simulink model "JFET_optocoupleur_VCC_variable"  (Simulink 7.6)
settings: Solver=ode15s  StartTime=0.0  StopTime=10.0  RelTol=1e-3
StopFcn:
  | close all, clc
  | load ID_Vcc_Variable.mat
  | delete *.mat
  | plotyy(x(1,:),x(2,:), x(1,:),x(3,:))
  | grid
  | title('Courant de drain ID et alimentation variable')
  | xlabel('temps')
libraries: fl_lib x10, elec_lib x5, nesl_utility x4

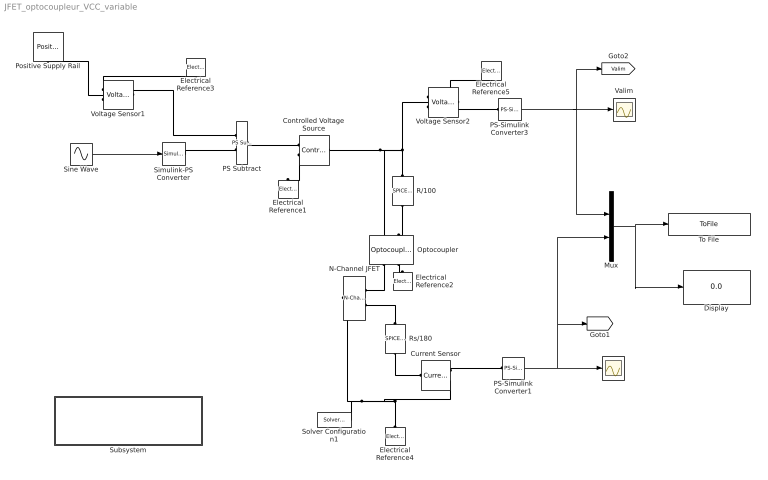
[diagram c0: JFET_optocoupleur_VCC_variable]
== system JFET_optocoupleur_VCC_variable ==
  Controlled Voltage Source : fl_lib/Electrical/Electrical Sources/Controlled Voltage Source  DialogController=NetworkEngine.DynNeDlgSource  SystemSampleTime=-1  i_Log=off  v_Log=off  LocalVarNames=|i|v  LocalVarDescs=|i|v  LocalVarLogging=[0 0]
  Current Sensor : fl_lib/Electrical/Electrical Sensors/Current Sensor  DialogController=NetworkEngine.DynNeDlgSource  SystemSampleTime=-1  i1_Log=off  v1_Log=off  LocalVarNames=|i1|v1  LocalVarDescs=|i1|v1  LocalVarLogging=[0 0]
  Display : Display
  Electrical Reference{1..5} (5 alike) : fl_lib/Electrical/Electrical Elements/Electrical Reference  DialogController=NetworkEngine.DynNeDlgSource  SystemSampleTime=-1  i_Log=off  LocalVarNames=|i  LocalVarDescs=|i  LocalVarLogging=[]
  I : Scope
  Mux : Mux  Inputs=2
  N-Channel JFET : elec_lib/Semiconductor Devices/N-Channel JFET  DialogController=NetworkEngine.DynNeDlgSource  SystemSampleTime=-1  parameterization=1  Igss=-1 nA  Idss=17 mA  Idss_v="[  0 15 ] V"  ssig="[  3e+03 10 ] uS"  ssig_v="[  0 15 ] V"  Beta=1e-04 A/V^2  IS=1e-14 A  Tmeas=25 C  Vt0=-2 V  Lchannel=0 1/V  RS=0.1 Ohm  RD=0.1 Ohm  C_param=1  C_GS=3 pF  C_GD=1.5 pF  C_iss=4.5 pF  C_rss=1.5 pF  LocalVarLogging=[]
  Optocoupler : elec_lib/Semiconductor Devices/Optocoupler  DialogController=NetworkEngine.DynNeDlgSource  SystemSampleTime=-1  CTR=0.2  prmExp=1  I12="[  0.001 0.015 ] A"  V12="[  0.9 1.05 ] V"  RS=0.1 Ohm  IS=1e-10 A  Tmeas=25 C  ec=2  C_param=1  CJ0=5 pF  VJ=1 V  Mgrad=0.5  Vvec="[  0.1 10 100 ] V"  Cvec="[  3.5 1 0.4 ] pF"  FC=0.5  LocalVarLogging=[]
  PS Subtract : fl_lib/Physical Signals/Functions/PS Subtract  DialogController=NetworkEngine.DynNeDlgSource  SystemSampleTime=-1  LocalVarLogging=[]
  PS-Simulink Converter1 : nesl_utility/PS-Simulink Converter  DialogController=NetworkEngine.DynNeUtilDlgSource  SystemSampleTime=-1  PhysicalDomain=network_engine_domain  LeftPortType=input  RightPortType=output  SubClassName=ps_output  Unit=1  AffineConversion=off
  PS-Simulink Converter3 : nesl_utility/PS-Simulink Converter  DialogController=NetworkEngine.DynNeUtilDlgSource  SystemSampleTime=-1  PhysicalDomain=network_engine_domain  LeftPortType=input  RightPortType=output  SubClassName=ps_output  Unit=1  AffineConversion=off
  Positive Supply Rail : elec_lib/Sources/Positive Supply Rail  DialogController=NetworkEngine.DynNeDlgSource  SystemSampleTime=-1  v0=15 V  current_Log=off  voltage_Log=off  power_Log=off  LocalVarNames=|current|voltage|power  LocalVarDescs=|Current (A)|Voltage (V)|Power (W)  LocalVarLogging=[0 0 0]
  R/100 : elec_lib/Additional Components/SPICE-Compatible Components/Passive Devices/SPICE Resistor  DialogController=NetworkEngine.DynNeDlgSource  SystemSampleTime=-1  SCALE=1  R_param=1  R=100 Ohm  RSH=0 Ohm  LENGTH=1e-06 m  WIDTH=1e-06 m  NARROW=0 m  T_param=1  TC1=0 1/K  TC2=0 1/K^2  TOFFSET=0 K  TFIXED=300.15 K  TMEAS=300.15 K  LocalVarLogging=[]
  Rs/180 : elec_lib/Additional Components/SPICE-Compatible Components/Passive Devices/SPICE Resistor  DialogController=NetworkEngine.DynNeDlgSource  SystemSampleTime=-1  SCALE=1  R_param=1  R=180 Ohm  RSH=0 Ohm  LENGTH=1e-06 m  WIDTH=1e-06 m  NARROW=0 m  T_param=1  TC1=0 1/K  TC2=0 1/K^2  TOFFSET=0 K  TFIXED=300.15 K  TMEAS=300.15 K  LocalVarLogging=[]
  Simulink-PS Converter : nesl_utility/Simulink-PS Converter  DialogController=NetworkEngine.DynNeUtilDlgSource  SystemSampleTime=-1  PhysicalDomain=network_engine_domain  LeftPortType=input  RightPortType=output  SubClassName=ps_input  Unit=1  AffineConversion=off  InputFilterTimeConstant=.001  UdotUserProvided=0
  Sine Wave : Sin  Amplitude=2  SampleTime=0
  Solver Configuration1 : nesl_utility/Solver Configuration  DialogController=NetworkEngine.DynNeUtilDlgSource  SystemSampleTime=-1  PhysicalDomain=network_engine_domain  LeftPortType=input  RightPortType=generic  SubClassName=solver  Accelerate=off  Profile=off  ResidualTolerance=1e-9  MaxNonlinIter=12  MaxModeIter=2  DoFixedCost=off  UseLocalSampling=off  DoDC=off  LinearAlgebra=Sparse  LocalSolverSampleTime=.001  LocalSolverChoice=NE_BACKWARD_EULER_ADVANCER  UseLocalSolver=off
  Subsystem : Subsystem
  To File : ToFile  Filename=ID_Vcc_Variable  MatrixName=x
  Valim : Scope
  Voltage Sensor1 : fl_lib/Electrical/Electrical Sensors/Voltage Sensor  DialogController=NetworkEngine.DynNeDlgSource  SystemSampleTime=-1  i1_Log=off  v1_Log=off  LocalVarNames=|i1|v1  LocalVarDescs=|i1|v1  LocalVarLogging=[0 0]
  Voltage Sensor2 : fl_lib/Electrical/Electrical Sensors/Voltage Sensor  DialogController=NetworkEngine.DynNeDlgSource  SystemSampleTime=-1  i1_Log=off  v1_Log=off  LocalVarNames=|i1|v1  LocalVarDescs=|i1|v1  LocalVarLogging=[0 0]
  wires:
  Sine Wave/1 -> Simulink-PS Converter/1
  PS-Simulink Converter1/1 -> I/1, [I], Mux/2
  PS-Simulink Converter3/1 -> Valim/1, [Valim], Mux/1
  Mux/1 -> To File/1, Display/1
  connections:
  N-Channel JFET/LConn1 -- Solver Configuration1/RConn1 -- Electrical Reference4/LConn1 -- Current Sensor/RConn2
  Rs/180/LConn1 -- N-Channel JFET/RConn2
  Optocoupler/LConn1 -- Controlled Voltage Source/LConn1 -- R/100/LConn1 -- Voltage Sensor2/LConn1
  Optocoupler/RConn1 -- N-Channel JFET/RConn1
  Optocoupler/RConn2 -- Electrical Reference2/LConn1
  R/100/RConn1 -- Optocoupler/LConn2
  Simulink-PS Converter/RConn1 -- PS Subtract/LConn2
  PS Subtract/RConn1 -- Controlled Voltage Source/RConn1
  Rs/180/RConn1 -- Current Sensor/LConn1
  Current Sensor/RConn1 -- PS-Simulink Converter1/LConn1
  Controlled Voltage Source/RConn2 -- Electrical Reference1/LConn1
  Voltage Sensor2/RConn1 -- PS-Simulink Converter3/LConn1
  Voltage Sensor2/RConn2 -- Electrical Reference5/LConn1
  Voltage Sensor1/RConn1 -- PS Subtract/LConn1
  Voltage Sensor1/LConn1 -- Positive Supply Rail/RConn1
  Voltage Sensor1/RConn2 -- Electrical Reference3/LConn1

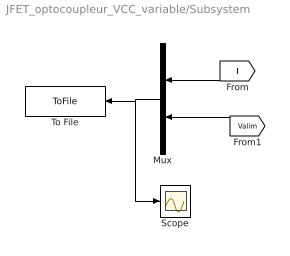
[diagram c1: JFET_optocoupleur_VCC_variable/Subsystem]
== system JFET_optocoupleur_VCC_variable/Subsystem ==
  Mux : Mux  Inputs=2
  Scope : Scope
  To File : ToFile  Filename=I_Valim  MatrixName=x
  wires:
  [I] -> Mux/1
  [Valim] -> Mux/2
  Mux/1 -> To File/1, Scope/1
